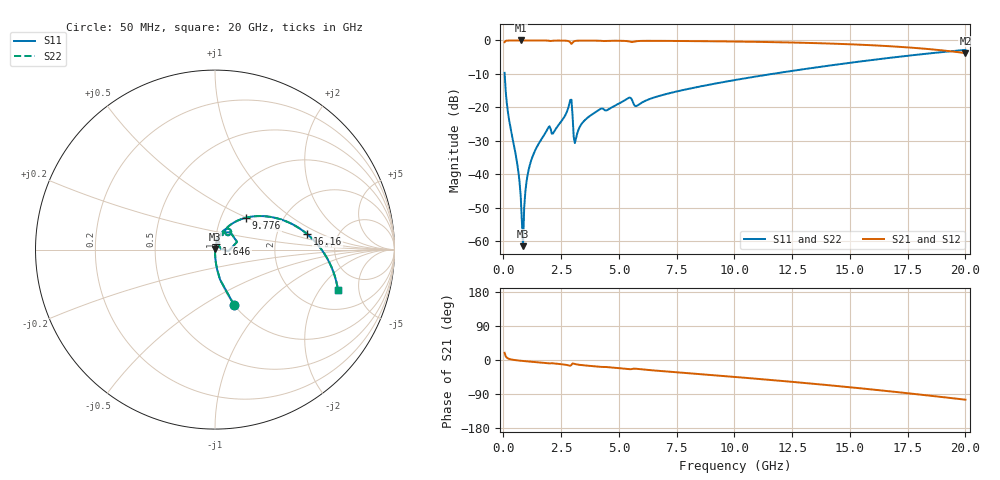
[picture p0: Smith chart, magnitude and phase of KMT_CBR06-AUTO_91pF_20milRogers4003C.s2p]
! Data measured by Modelithics Inc. support@modelithics.com 813-866-6335
! KEMET CBR06-AUTO 91pF, Pad Width= 0.851mm, Pad Length= 0.64mm, Pad Gap= 0.62mm, 20mil Rogers 4003C substrate Data, January 2022
# hz S ma R 50
! 2 Port Network Data from SP1.SP block
! freq  magS11  angS11  magS21  angS21  magS12  angS12  magS22  angS22
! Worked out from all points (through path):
!   401 points, 50 MHz to 20 GHz, reference 50 ohm
!   highest |S21| = 0.00 dB at 748.2 MHz (marker M1); lowest = -3.8 dB at 20 GHz (marker M2)
!   group delay of S21, straight-line fit = 14.5 ps
!   lowest |S11| = -61.5 dB at 848 MHz (marker M3), VSWR 1.00, Z = 50.1 + j0.0678 ohm
!   |S11| at or under -10 dB: 52.75 MHz to 11.64 GHz (11.59 GHz wide, 198 % of centre)
!   |S22| runs from -61.5 to -2.8 dB; largest |S21 - S12| = 0
!   S11 on the Smith chart (normalised r, x): 50 MHz: 1.00, -0.69; 1.646 GHz: 1.01, +0.07; 9.776 GHz: 1.31, +0.50; 16.16 GHz: 2.98, +0.71; 20 GHz: 3.18, -3.01
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5e7  0.3279 -71.0  0.9444 19.0  0.9444 19.0  0.3279 -71.0
2.495e8  0.06352 -86.9  0.9977 2.9  0.9977 2.9  0.06352 -86.9
5.98625e8  0.01421 -89.4  0.9995 -1.0  0.9995 -1.0  0.01421 -89.4
7.4825e8  0.004618 -86.5  0.9995 -2.0  0.9995 -2.0  0.004618 -86.5
8.48e8  0.0008421 53.5  0.9995 -2.6  0.9995 -2.6  0.0008421 53.5
8.97875e8  0.003168 78.3  0.9995 -2.9  0.9995 -2.9  0.003168 78.3
1.14725e9  0.01396 83.4  0.9993 -4.3  0.9993 -4.3  0.01396 83.4
1.646e9  0.03351 81.4  0.9984 -6.9  0.9984 -6.9  0.03351 81.4
1.94525e9  0.04998 73.5  0.992 -8.7  0.992 -8.7  0.04998 73.5
2.194625e9  0.04346 74.2  0.9939 -9.1  0.9939 -9.1  0.04346 74.2
2.843e9  0.1092 61.8  0.9687 -14.7  0.9687 -14.7  0.1092 61.8
3.14225e9  0.03447 58.0  0.9872 -11.3  0.9872 -11.3  0.03447 58.0
3.391625e9  0.05714 72.5  0.9943 -13.5  0.9943 -13.5  0.05714 72.5
5.386625e9  0.1366 58.9  0.9736 -24.0  0.9736 -24.0  0.1366 58.9
5.785625e9  0.1058 56.7  0.9761 -23.4  0.9761 -23.4  0.1058 56.7
6.73325e9  0.1478 60.1  0.9857 -28.7  0.9857 -28.7  0.1478 60.1
9.775625e9  0.2475 45.8  0.9657 -43.5  0.9657 -43.5  0.2475 45.8
1.0025e10  0.2562 44.6  0.9633 -44.7  0.9633 -44.7  0.2562 44.6
1.336662e10  0.3878 26.7  0.9154 -62.4  0.9154 -62.4  0.3878 26.7
1.615962e10  0.5205 9.6  0.8407 -79.0  0.8407 -79.0  0.5205 9.6
1.670825e10  0.5487 5.9  0.8205 -82.5  0.8205 -82.5  0.5487 5.9
2e10  0.7219 -18.3  0.6472 -104.7  0.6472 -104.7  0.7219 -18.3
